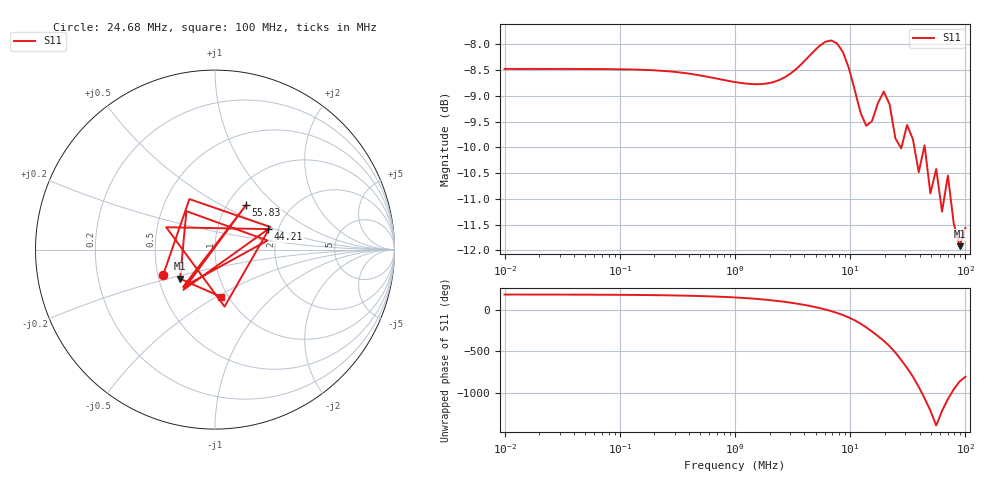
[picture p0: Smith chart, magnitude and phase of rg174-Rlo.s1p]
! ListType=Log
!!RG174 24.9f Rlo
# MHz S RI R 50
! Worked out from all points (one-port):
!   80 points, 10 kHz to 100 MHz, reference 50 ohm
!   lowest |S11| = -11.9 dB at 89 MHz (marker M1), VSWR 1.68, Z = 32.2 - j11.2 ohm
!   |S11| at or under -10 dB: 27.39 MHz to 27.9 MHz (514.7 kHz wide, 1.86 % of centre); 36.08 MHz to 43.85 MHz (7.776 MHz wide, 19.5 % of centre); 44.44 MHz to end of sweep
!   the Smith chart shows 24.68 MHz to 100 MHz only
!   S11 on the Smith chart (normalised r, x): 24.68 MHz: 0.53, -0.17; 44.21 MHz: 1.77, +0.45; 55.83 MHz: 1.22, +0.66; 100 MHz: 0.92, -0.52
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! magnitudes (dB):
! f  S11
! 10 kHz  -8.5
! 32.09 kHz  -8.5
! 103 kHz  -8.5
! 330.4 kHz  -8.5
! 1.06 MHz  -8.7
! 2.134 MHz  -8.7
! 3.401 MHz  -8.5
! 6.846 MHz  -7.9
! 8.644 MHz  -8.2
! 10.91 MHz  -8.9
! 12.26 MHz  -9.3
! 13.78 MHz  -9.6
! 15.48 MHz  -9.5
! 19.55 MHz  -8.9
! 21.97 MHz  -9.2
! 24.68 MHz  -9.8
! 27.74 MHz  -10.0
! 31.17 MHz  -9.6
! 35.02 MHz  -9.8
! 39.35 MHz  -10.5
! 44.21 MHz  -10.0
! 49.68 MHz  -10.9
! 55.83 MHz  -10.4
! 62.73 MHz  -11.2
! 70.49 MHz  -10.5
! 79.2 MHz  -11.5
! 89 MHz  -11.9
! 100 MHz  -11.6
